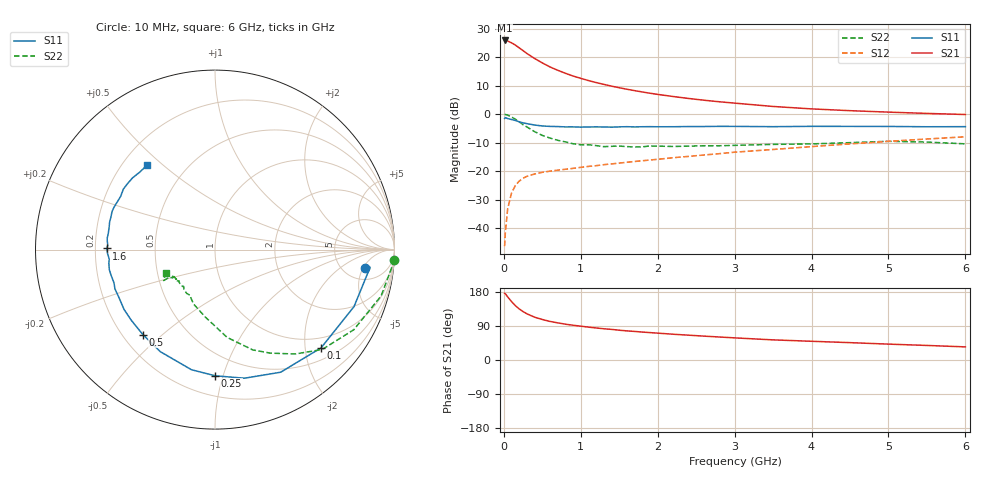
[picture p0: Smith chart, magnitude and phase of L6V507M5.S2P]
!  INFINEON TECHNOLOGIES Small Signal Semiconductors
! BFR380L3 , Si-NPN RF-Transistor in TSLP-3-1
!  Vce=0.5 V,  Ic=7.5 mA
! Common Emitter S-Parameters:  07. March 2005
#  GHz  S  MA  R  50
! f  S11  S21  S12  S22
! GHz  Mag  Ang  Mag  Ang  Mag  Ang  Mag  Ang
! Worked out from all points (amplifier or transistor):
!   36 points, 10 MHz to 6 GHz, reference 50 ohm
!   highest |S21| = 25.9 dB at 10 MHz (marker M1)
!   |S21| within 3 dB of that: start of sweep to 220.1 MHz
!   unconditionally stable (mu >= 1): 1.976 GHz to 5.78 GHz
!   at 250 MHz: K = 0.24, MSG = 22.4 dB, |S12| = -22.5 dB
!   at 1.4 GHz: K = 0.88, MSG = 13.7 dB, |S12| = -17.5 dB
!   at 6 GHz: K = 1.00, MSG = 3.9 dB, |S12| = -7.9 dB
!   S11 on the Smith chart (normalised r, x): 10 MHz: 7.73, -5.39; 100 MHz: 0.75, -2.35; 250 MHz: 0.34, -0.94; 500 MHz: 0.28, -0.43; 1.6 GHz: 0.25, +0.00; 6 GHz: 0.30, +0.44
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0.01  0.8403 -7.0  19.75 175.6  0.0048 84.5  1 -3.2
0.02  0.87 -6.5  19.64 174.8  0.0085 85.2  0.9865 -6.6
0.05  0.8371 -22.3  19.26 166.5  0.0219 79.7  0.9608 -15.6
0.1  0.8056 -42.8  17.95 154.2  0.0413 68.7  0.8928 -30.0
0.15  0.775 -61.8  16.36 143.4  0.0559 60.7  0.8163 -43.0
0.2  0.7351 -77.1  14.62 134.7  0.0668 54.6  0.7333 -52.5
0.25  0.7031 -89.9  13.08 127.8  0.075 49.3  0.6531 -62.0
0.3  0.682 -101.1  11.65 121.9  0.0809 46.5  0.5968 -69.4
0.4  0.6451 -118.2  9.524 113.0  0.089 42.1  0.4934 -82.2
0.5  0.621 -130.3  7.961 106.9  0.0951 40.1  0.4239 -90.3
0.6  0.6104 -139.8  6.762 101.8  0.0999 39.4  0.3807 -98.0
0.7  0.6065 -146.7  5.913 98.0  0.1038 39.5  0.3477 -105.0
0.9  0.5988 -158.6  4.682 91.7  0.1117 40.5  0.3024 -116.2
1.1  0.5962 -166.0  3.899 86.7  0.1209 42.4  0.2906 -123.0
1.4  0.5915 -174.9  3.109 80.8  0.1337 45.1  0.2726 -131.0
1.6  0.6033 179.4  2.743 76.8  0.143 46.4  0.2694 -138.2
2.2  0.6022 168.7  2.045 68.0  0.1718 50.7  0.2709 -142.3
2.8  0.6115 159.6  1.654 60.7  0.2025 53.6  0.2789 -147.9
3.5  0.6035 150.6  1.367 53.1  0.2399 54.3  0.2947 -148.3
4.5  0.6106 143.4  1.153 45.8  0.301 55.3  0.3163 -148.9
5.5  0.6017 134.2  1.032 38.4  0.3666 53.1  0.3237 -150.8
6  0.6039 128.7  0.987 34.6  0.4009 51.5  0.3012 -154.9
